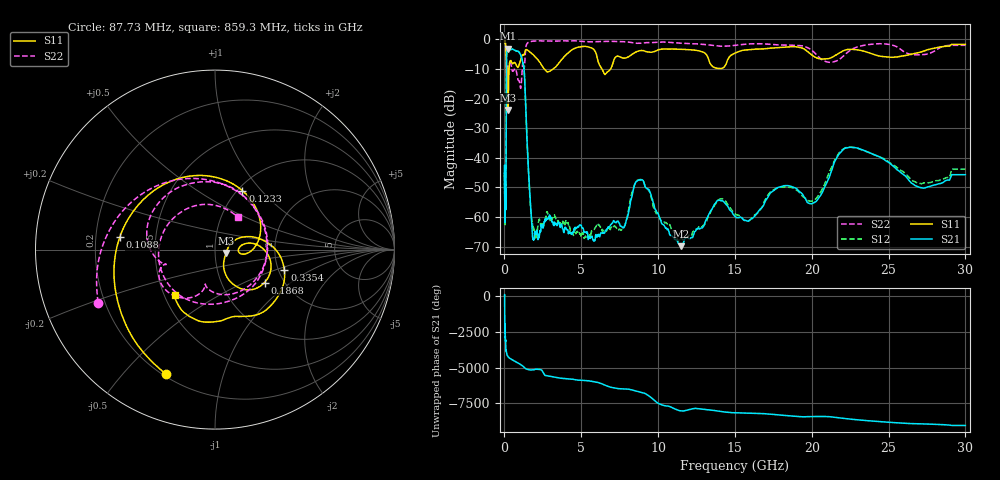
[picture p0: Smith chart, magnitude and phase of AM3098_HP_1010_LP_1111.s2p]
! Date/Time: Thu, Feb 28, 2019 8:42 AM
! Network Analyzer: Agilent Technologies E8364B Rev: A.07.50.67
! Sweep from 0.010 to 30.000 GHz, 1601 Points, Sweep Type: LOG
! Power Supply: 5.022 V, 0.002 A
# Hz S DB R 50
!freq MagS11 AngS11 MagS21 AngS21 MagS12 AngS12 MagS22 AngS22
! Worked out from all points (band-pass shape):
!   1601 points, 10 MHz to 30 GHz, reference 50 ohm
!   highest |S21| = -3.15 dB at 256 MHz (marker M1); lowest = -69.8 dB at 11.48 GHz (marker M2)
!   |S21| within 3 dB of the highest: 133.8 MHz to 1.114 GHz (979.8 MHz wide, 157 % of centre)
!   lowest |S11| = -23.8 dB at 241.1 MHz (marker M3), VSWR 1.14, Z = 56.5 - j2.11 ohm
!   |S11| at or under -10 dB: 193.2 MHz to 300.3 MHz (107.1 MHz wide, 43.4 % of centre); 2.599 GHz to 3.169 GHz (569.2 MHz wide, 19.7 % of centre); 6.347 GHz to 6.906 GHz (558.4 MHz wide, 8.43 % of centre)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
!   |S22| runs from -16.5 to -0.5 dB; largest |S21 - S12| = 0.013
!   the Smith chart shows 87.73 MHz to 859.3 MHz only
!   S11 on the Smith chart (normalised r, x): 87.73 MHz: 0.21, -0.66; 108.8 MHz: 0.30, +0.06; 123.3 MHz: 1.05, +0.80; 186.8 MHz: 1.60, -0.66; 335.4 MHz: 2.15, -0.59; 859.3 MHz: 0.57, -0.32
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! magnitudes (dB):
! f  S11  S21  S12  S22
! 10 MHz  -0.3  -45.2  -45.8  -0.6
! 38.04 MHz  -0.4  -59.1  -59.9  -1.0
! 57.34 MHz  -1.0  -52.0  -49.6  -1.5
! 87.73 MHz  -2.5  -55.7  -55.4  -2.9
! 108.8 MHz  -5.4  -29.6  -29.9  -6.9
! 123.3 MHz  -8.8  -11.2  -11.2  -10.9
! 144.7 MHz  -17.7  -4.7  -4.7  -13.8
! 186.8 MHz  -9.6  -3.7  -3.7  -9.0
! 241.1 MHz  -23.8  -3.2  -3.1  -10.9
! 256 MHz  -19.0  -3.2  -3.1  -10.6
! 335.4 MHz  -7.9  -3.4  -3.4  -7.9
! 550.5 MHz  -8.1  -3.4  -3.3  -10.7
! 859.3 MHz  -9.5  -4.0  -3.9  -13.1
! 1.263 GHz  -5.3  -9.4  -9.4  -9.9
! 1.802 GHz  -4.9  -64.6  -61.4  -0.6
! 2.084 GHz  -6.3  -64.9  -66.2  -0.5
! 7.926 GHz  -6.2  -61.1  -61.3  -0.8
! 8.893 GHz  -3.8  -47.4  -47.3  -1.3
! 11.48 GHz  -3.3  -69.8  -67.4  -1.3
! 20.1 GHz  -5.6  -55.3  -54.5  -4.1
! 22.56 GHz  -3.4  -36.4  -36.4  -3.5
! 30 GHz  -1.7  -45.7  -43.8  -2.0
